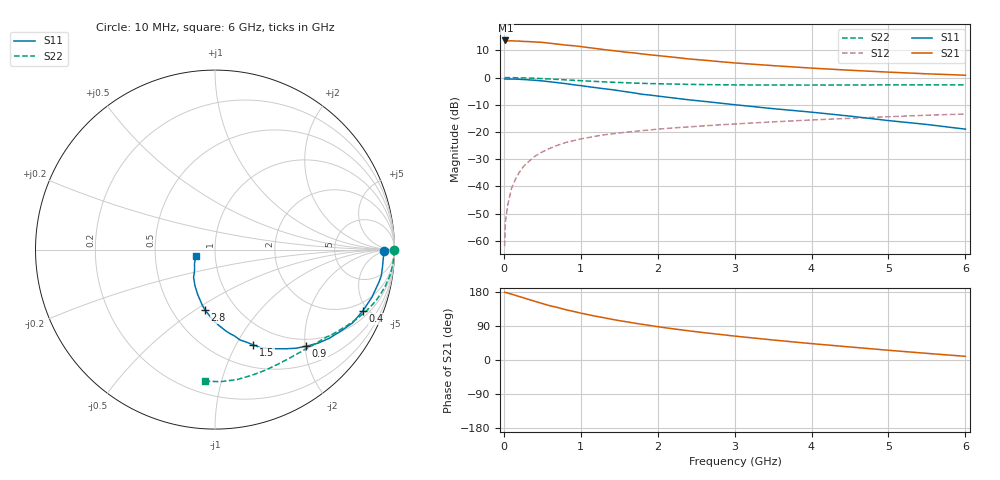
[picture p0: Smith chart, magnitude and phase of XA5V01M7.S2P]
! SIEMENS Discrete & RF Semiconductors
! BFY180
! Si NPN RF Bipolar Junction Transistor in MICRO-X
! VCE = 5 V  IC = 1.7 mA
! Common Emitter S-Parameters:  May  1997
# GHz  S  MA  R  50
!  f  S11  S21  S12  S22
! GHz  MAG  ANG  MAG  ANG  MAG  ANG  MAG  ANG
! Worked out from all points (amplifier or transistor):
!   36 points, 10 MHz to 6 GHz, reference 50 ohm
!   highest |S21| = 13.6 dB at 20 MHz (marker M1)
!   |S21| within 3 dB of that: start of sweep to 1.208 GHz
!   unconditionally stable (mu >= 1): 3.238 GHz to end of sweep
!   at 250 MHz: K = 0.10, MSG = 23.1 dB, |S12| = -32.8 dB
!   at 1.4 GHz: K = 0.61, MSG = 15.3 dB, |S12| = -20.7 dB
!   at 6 GHz: K = 1.06, MAG = 5.6 dB, |S12| = -13.4 dB
!   S11 on the Smith chart (normalised r, x): 10 MHz: 32, -5; 400 MHz: 1.39, -4.63; 900 MHz: 0.85, -2.02; 1.5 GHz: 0.75, -1.18; 2.8 GHz: 0.72, -0.55; 6 GHz: 0.80, -0.06
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0.01  0.941 -0.6  4.753 178.9  0.0008 83.8  0.997 -0.2
0.02  0.9418 -1.1  4.806 178.2  0.0022 98.3  0.9971 -0.6
0.05  0.9389 -2.8  4.705 176.9  0.0045 86.3  0.9963 -1.5
0.1  0.9383 -5.9  4.741 173.7  0.0093 88.2  0.9963 -3.1
0.15  0.938 -8.9  4.684 170.7  0.0135 85.8  0.994 -4.7
0.25  0.9199 -14.5  4.614 164.5  0.0228 81.3  0.9882 -7.8
0.4  0.8916 -22.5  4.514 155.1  0.0356 75.8  0.9709 -12.0
0.5  0.8686 -28.0  4.429 149.0  0.0431 71.5  0.9559 -14.9
0.6  0.8359 -32.8  4.271 143.1  0.0503 68.9  0.9419 -17.4
0.8  0.7752 -42.3  3.953 132.9  0.0639 63.2  0.9084 -22.2
0.9  0.7399 -46.7  3.855 128.4  0.0691 60.3  0.892 -24.3
1.1  0.6801 -54.3  3.553 119.5  0.0792 56.3  0.8611 -28.2
1.3  0.6242 -61.9  3.27 111.6  0.0886 52.5  0.8345 -31.7
1.5  0.5727 -68.1  3.036 103.9  0.0959 49.4  0.8123 -34.9
1.8  0.4922 -77.4  2.714 94.1  0.1063 46.1  0.7837 -39.3
2.2  0.4231 -87.1  2.372 82.3  0.1188 41.9  0.7607 -44.8
2.6  0.3657 -95.3  2.089 72.2  0.1297 38.7  0.744 -49.9
2.8  0.3409 -99.3  1.966 67.7  0.1353 37.4  0.7383 -52.3
3.5  0.2685 -111.0  1.657 52.8  0.1537 32.4  0.7287 -60.9
4.5  0.1958 -127.5  1.363 34.4  0.1787 25.3  0.7296 -73.7
5.5  0.1375 -146.0  1.172 17.5  0.2035 17.7  0.7364 -87.5
6  0.1129 -161.7  1.105 9.7  0.2141 13.6  0.7355 -94.4
